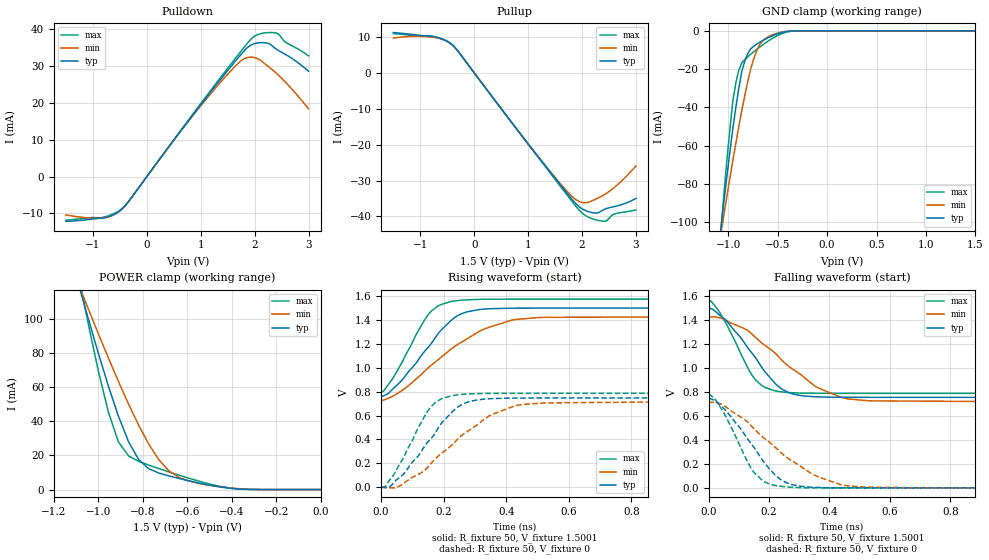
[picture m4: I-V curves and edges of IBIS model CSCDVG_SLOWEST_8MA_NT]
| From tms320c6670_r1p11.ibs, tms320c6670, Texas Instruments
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|   Model Cell CSCDVG_SLOWEST_8MA_NT
|SLOWEST_8MA
[Model]   CSCDVG_SLOWEST_8MA_NT
Model_type   I/O
Polarity   Non-Inverting
Enable   Active-Low
Cref =  4.0000pF
Rref =  100.0000M
Vref =  0V
Vmeas =  0.75
C_comp   1.5249p   1.4275p   1.6205p
|[mode_tieoffpin] SR0=1  SR1=1 I0=0 I1=0 I2=1
[Model Spec]
Vinl   0.6125   0.6125   0.6125
Vinh   0.9625   0.9625   0.9625
D_overshoot_high 1.95 1.95 1.95
D_overshoot_low -0.3 -0.3 -0.3
D_overshoot_time 1E-9 1E-9 1E-9
S_overshoot_high 1.575 1.575 1.575
S_overshoot_low 0 0 0
[Receiver Thresholds]
Reference_supply Pullup_ref
Threshold_sensitivity= 0.5
Tslew_ac= 5nS
Vinh_ac= +175mV
Vinh_dc= +100mV
Vinl_ac= -175mV
Vinl_dc= -100mV
Vth = 0.75
Vth_max= 0.79
Vth_min= 0.71
[Pullup Reference] 1.5001   1.425   1.575
[Add Submodel]
|Submodel_name Mode
CSCDVG_NT Non-Driving
[Temperature Range]   25   105   -40
[Voltage Range]   1.5   1.425   1.575
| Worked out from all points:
|   slope of the pulldown table from 0 to 0.225 V, typ, clamps not added: 50.1 ohm
|   slope of the pullup table from 0 to 0.225 V, typ, clamps not added: 50.1 ohm
|   GND clamp passes 1 mA (typ) near -0.47 V on its own axis
|   POWER clamp passes 1 mA (typ) near -0.42 V on its own axis
|   rising waveform, R_fixture 50, V_fixture 1.5001: 20-80 % time 136ps typ, 208ps min, 98ps max; typ from 0.756 V to 1.5 V
|   rising waveform, R_fixture 50, V_fixture 0: 20-80 % time 132ps typ, 191ps min, 95.4ps max; typ from 0 V to 0.747 V
|   falling waveform, R_fixture 50, V_fixture 1.5001: 20-80 % time 135ps typ, 202ps min, 94.9ps max; typ from 1.5 V to 0.755 V
|   falling waveform, R_fixture 50, V_fixture 0: 20-80 % time 132ps typ, 207ps min, 92.7ps max; typ from 0.746 V to 0 V
[POWER_clamp]
|   voltage   I(typ)   I(min)   I(max)
-1.5V     321.7mA    260.6mA    415.9mA
-1.076V   114.2mA    115.8mA    116.9mA
-1.061V   107.2mA    110.9mA    107.1mA
-954.6mV  60.59mA    77.06mA    45.35mA
-909.2mV  42.85mA    63.21mA    27.81mA
-863.7mV  27.9mA     49.99mA    19.69mA
-818.2mV  17.49mA    37.63mA    16.52mA
-772.8mV  12.19mA    26.53mA    14.33mA
-681.9mV  7.985mA    10.89mA    10.33mA
-590.9mV  5.094mA    4.955mA    6.6mA
-363.7mV  298.5uA    465.2uA    297.6uA
0V        1.518nA    24.08nA    367.8pA
[Pulldown]
|   voltage   I(typ)   I(min)   I(max)
-1.5V     -12.15mA   -10.4mA    -11.83mA
-863.7mV  -11.34mA   -11.22mA   -11.25mA
-500mV    -9.267mA   -9.352mA   -9.148mA
-318.2mV  -6.354mA   -6.371mA   -6.385mA
1.046V    20.42mA    20.05mA    20.72mA
1.591V    30.47mA    29.26mA    31.18mA
1.818V    34.39mA    32.13mA    35.4mA
1.955V    35.92mA    32.45mA    37.67mA
2.091V    36.38mA    31.76mA    38.77mA
2.273V    36.08mA    29.69mA    39.15mA
2.364V    35.03mA    28.59mA    39.11mA
3V        28.64mA    18.41mA    32.82mA
[Pullup]
|   voltage   I(typ)   I(min)   I(max)
-1.5V     11.21mA    9.69mA     10.94mA
-818.2mV  10.23mA    9.978mA    10.29mA
-590.9mV  9.401mA    9.328mA    9.374mA
-409.1mV  7.828mA    7.781mA    7.859mA
1.227V    -24.14mA   -24.11mA   -24.35mA
1.727V    -33.63mA   -33.09mA   -34.13mA
1.909V    -36.81mA   -35.55mA   -37.6mA
2.046V    -38.25mA   -36.2mA    -39.57mA
2.227V    -39.04mA   -35.36mA   -40.83mA
2.409V    -38.05mA   -33.98mA   -41.36mA
2.591V    -37.29mA   -32.03mA   -39.38mA
3V        -34.98mA   -25.95mA   -38.2mA
[GND_clamp]
|   voltage   I(typ)   I(min)   I(max)
-1.5V     -310.1mA   -250.5mA   -402.5mA
-1.076V   -103.6mA   -106.2mA   -105.2mA
-1.046V   -89.81mA   -96.36mA   -86.02mA
-954.6mV  -51.22mA   -67.87mA   -36.88mA
-924.3mV  -40.08mA   -58.86mA   -27.29mA
-863.7mV  -21.24mA   -41.56mA   -16.73mA
-833.4mV  -15.8mA    -33.75mA   -15.03mA
-772.8mV  -9.345mA   -19.75mA   -12.19mA
-712.2mV  -6.928mA   -10.35mA   -9.704mA
-621.3mV  -4.261mA   -3.896mA   -6.225mA
-409.1mV  -337.1uA   -289.1uA   -618.9uA
1.5V      1.518nA    257.2nA    299pA
[Ramp]
| variable   typ   min   max
dV/dt_f   0.596016/0.19469535n   0.56432/0.3101823n   0.629272/0.14102085n
dV/dt_r  0.6013584/0.19239092n 0.57508648/0.29752883n 0.63081544/0.1406002n
R_load = 50
[Rising Waveform]
R_fixture = 50
V_fixture = 1.5001
V_fixture_min = 1.425
V_fixture_max = 1.575
|   time   V(typ)   V(min)   V(max)
0s        755.9mV    721.6mV    789.3mV
35.49ps   817.7mV    760.2mV    904.4mV
62.87ps   885.6mV    803mV      1.027V
149.8ps   1.17V      998.8mV    1.443V
178.6ps   1.274V     1.061V     1.512V
221.3ps   1.391V     1.151V     1.554V
273.4ps   1.468V     1.241V     1.569V
326.2ps   1.491V     1.321V     1.573V
428.6ps   1.499V     1.404V     1.575V
1.283ns   1.5V       1.425V     1.575V
[Rising Waveform]
R_fixture = 50
V_fixture = 0
V_fixture_min = 0
V_fixture_max = 0
|   time   V(typ)   V(min)   V(max)
0s        0V         0V         0V
25.42ps   0V         -5.021mV   54.37mV
69.9ps    105.4mV    28.32mV    239.7mV
153.8ps   392.2mV    182.2mV    656.3mV
186.7ps   513.3mV    270.6mV    731.7mV
227.1ps   630.7mV    355.1mV    766.8mV
273.1ps   709mV      462.7mV    780.1mV
345.9ps   740.4mV    597.8mV    785.2mV
454.4ps   746.6mV    693.4mV    786.1mV
1.291ns   747.3mV    712.8mV    786.3mV
[Falling Waveform]
R_fixture = 50
V_fixture = 1.5001
V_fixture_min = 1.425
V_fixture_max = 1.575
|   time   V(typ)   V(min)   V(max)
0s        1.499V     1.424V     1.575V
33.01ps   1.449V     1.421V     1.48V
59.02ps   1.395V     1.395V     1.368V
152.3ps   1.098V     1.263V     910.9mV
180.5ps   989.3mV    1.2V       847.3mV
218.6ps   876.3mV    1.129V     810.4mV
275.3ps   786.6mV    995.1mV    793.7mV
351.6ps   760.1mV    849.6mV    789.3mV
462.4ps   755.6mV    741.7mV    788.7mV
1.283ns   755.2mV    720.6mV    788.5mV
[Falling Waveform]
R_fixture = 50
V_fixture = 0
V_fixture_min = 0
V_fixture_max = 0
|   time   V(typ)   V(min)   V(max)
0s        746.3mV    712.1mV    785.4mV
25.7ps    715.6mV    711.7mV    726.6mV
50.56ps   662.3mV    687.6mV    625.4mV
148.6ps   344mV      497.2mV    133.8mV
179.2ps   228.6mV    423.6mV    59.31mV
216.4ps   117.8mV    348.9mV    21.84mV
281.3ps   24.07mV    217.9mV    4.324mV
356ps     4.058mV    99.56mV    0V
455.4ps   0V         18.18mV    0V
1.291ns   0V         0V         0V
